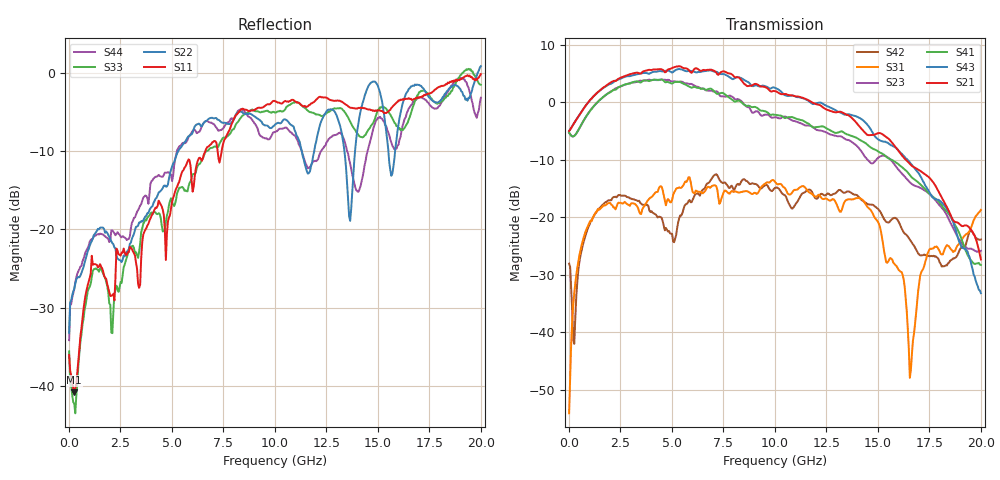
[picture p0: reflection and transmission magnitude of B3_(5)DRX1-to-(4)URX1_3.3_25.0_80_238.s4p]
!Agilent Technologies,N5225A,MY51451112,A.09.50.13
!Agilent N5225A: A.09.50.13
!Date: Sunday, March 12, 2017 05:23:14
!Correction: S11(Full 4 Port(1,2,3,4))
!S12(Full 4 Port(1,2,3,4))
!S13(Full 4 Port(1,2,3,4))
!S14(Full 4 Port(1,2,3,4))
!S21(Full 4 Port(1,2,3,4))
!S22(Full 4 Port(1,2,3,4))
!S23(Full 4 Port(1,2,3,4))
!S24(Full 4 Port(1,2,3,4))
!S31(Full 4 Port(1,2,3,4))
!S32(Full 4 Port(1,2,3,4))
!S33(Full 4 Port(1,2,3,4))
!S34(Full 4 Port(1,2,3,4))
!S41(Full 4 Port(1,2,3,4))
!S42(Full 4 Port(1,2,3,4))
!S43(Full 4 Port(1,2,3,4))
!S44(Full 4 Port(1,2,3,4))
!S4P File: Measurements: <S11,S12,S13,S14>,
!<S21,S22,S23,S24>,
!<S31,S32,S33,S34>,
!<S41,S42,S43,S44>:
# Hz S  dB  R 50
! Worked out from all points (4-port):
!   401 points, 10 MHz to 20 GHz, reference 50 ohm
!   strongest paths, dB at 10 MHz, 5.008 GHz, 10.01 GHz, 15 GHz, 20 GHz:
!     S21: -5.0, 5.9, 1.9, -5.4, -27.3
!     S43: -5.0, 5.2, 2.5, -6.4, -33.2
!     S41: -5.3, 3.2, -2.2, -8.5, -28.3
!     S23: -5.3, 3.6, -2.6, -9.7, -25.8
!     S31: -54.1, -17.0, -13.9, -20.8, -18.7
!     S42: -28.1, -22.9, -14.9, -18.5, -23.9
!   lowest |S11| = -40.8 dB at 259.9 MHz (marker M1), VSWR 1.02, Z = 50.3 - j0.87 ohm
!   |S11| at or under -10 dB: start of sweep to 6.626 GHz; 7.22 GHz to 7.416 GHz (196.1 MHz wide, 2.68 % of centre)
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1e7  -36.07 -38.6  -62.42 118.2  -53.20 15.5  -77.57 118.4
     -5.01 1.9  -33.23 40.0  -5.33 -179.4  -27.99 38.0
     -54.07 28.4  -63.76 122.4  -35.60 -44.8  -65.44 173.8
     -5.32 -179.4  -28.07 38.1  -4.99 2.1  -34.16 45.1
2.59875e8  -40.82 -72.1  -49.96 57.4  -33.09 94.8  -50.76 53.9
           -3.60 7.1  -27.61 -132.0  -5.85 -177.9  -41.70 -161.9
           -33.19 95.2  -49.69 58.5  -42.30 -77.9  -50.80 54.9
           -5.85 -178.7  -42.01 -171.4  -3.58 6.3  -27.62 -137.8
2.858575e9  -22.92 149.6  -39.07 -35.9  -17.70 54.9  -37.98 -46.2
            4.73 -90.2  -22.79 157.7  3.19 82.9  -16.35 42.1
            -17.79 54.6  -38.58 -29.2  -23.15 125.7  -37.58 -37.7
            3.19 73.1  -16.52 41.5  4.52 -98.3  -21.28 138.6
4.957525e9  -17.37 96.4  -42.32 -31.9  -16.78 29.5  -37.76 -19.6
            5.85 172.1  -12.39 149.9  3.62 -23.7  -24.42 28.6
            -17.40 21.7  -40.09 3.3  -16.04 108.5  -34.99 6.6
            3.28 -39.3  -22.85 39.1  5.25 159.1  -13.05 116.1
7.956025e9  -6.25 41.4  -32.71 -101.9  -16.54 7.8  -31.96 -122.0
            4.70 22.1  -6.16 88.5  0.89 -165.1  -14.40 50.6
            -15.52 6.3  -29.94 -102.3  -7.22 64.9  -30.65 -132.8
            0.37 169.9  -14.88 48.0  3.99 10.8  -5.96 42.9
1.155422e10  -4.32 -6.1  -37.40 -117.7  -14.70 -22.4  -40.09 -137.0
             0.46 -133.6  -12.61 85.3  -4.05 40.8  -15.37 37.0
             -15.24 -23.4  -33.53 -122.9  -4.74 10.5  -34.14 -151.8
             -3.61 3.0  -15.36 42.5  0.39 -158.6  -11.87 25.4
2e10  -0.17 -114.2  -32.99 62.8  -18.75 121.1  -35.52 21.6
      -27.32 -164.2  0.85 17.1  -25.84 20.8  -23.91 101.9
      -18.72 121.1  -33.99 40.3  -1.53 -87.7  -35.28 -7.8
      -28.30 -27.8  -23.86 102.9  -33.19 165.3  -3.18 -136.7
